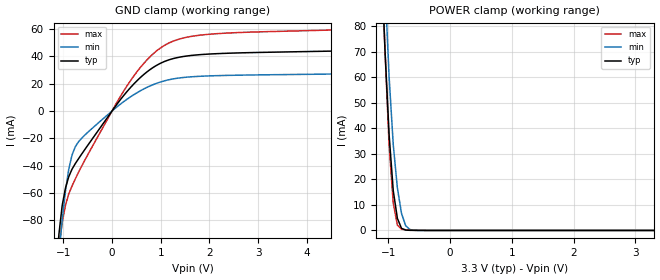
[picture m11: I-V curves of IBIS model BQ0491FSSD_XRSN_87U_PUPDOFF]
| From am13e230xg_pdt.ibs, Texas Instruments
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|   Model BQ0491FSSD_XRSN_87U_PUPDOFF
[Model] BQ0491FSSD_XRSN_87U_PUPDOFF
Model_type Input
Polarity   Non-Inverting
Enable   Active-High
Vinl =  0.990V
Vinh =  2.310V
C_comp_power_clamp   0.230pF   0.207pF   0.251pF
[Model Spec]
Vinh   2.310V   2.079V   2.541V
Vinl   0.990V   0.891V   1.089V
[Temperature Range]   25.000   0.155k   -40.000
[Voltage Range]   3.300V   2.970V   3.630V
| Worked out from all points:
|   GND clamp passes 1 mA (typ) near -0.02 V on its own axis
|   POWER clamp passes 1 mA (typ) near -0.79 V on its own axis
[GND_clamp]
|Voltage   I(typ)   I(min)   I(max)
-3.3V     -1.509A    -1.199A    -2.021A
-1.089V   -89.98mA   -104.5mA   -99.46mA
-1.022V   -69.04mA   -79.67mA   -81.46mA
-955mV    -56.37mA   -58.56mA   -68.94mA
-888mV    -48.09mA   -42.63mA   -60.66mA
-821mV    -42.55mA   -32.25mA   -54.94mA
-687mV    -34.88mA   -22.46mA   -44.8mA
385mV     17.4mA     10.52mA    22.49mA
787mV     30.49mA    18.46mA    39.95mA
1.189V    37.69mA    23.05mA    50.13mA
2.261V    42.13mA    25.99mA    56.84mA
6.6V      45.19mA    27.91mA    61.13mA
[POWER_clamp]
|Voltage   I(typ)   I(min)   I(max)
-3.3V     1.754A     1.982A     1.894A
-1.122V   110.7mA    138.8mA    115.5mA
-1.055V   70.74mA    96.23mA    70.78mA
-988mV    37.52mA    60.27mA    33.45mA
-921mV    15.62mA    33.67mA    10.79mA
-854mV    4.739mA    16.67mA    2.07mA
-787mV    816.2uA    6.677mA    461.1uA
-720mV    142.1uA    1.876mA    284.8uA
-653mV    56.07uA    385.4uA    208.9uA
-586mV    33.33uA    60.07uA    150.6uA
3.3V      0A         0A         0A
